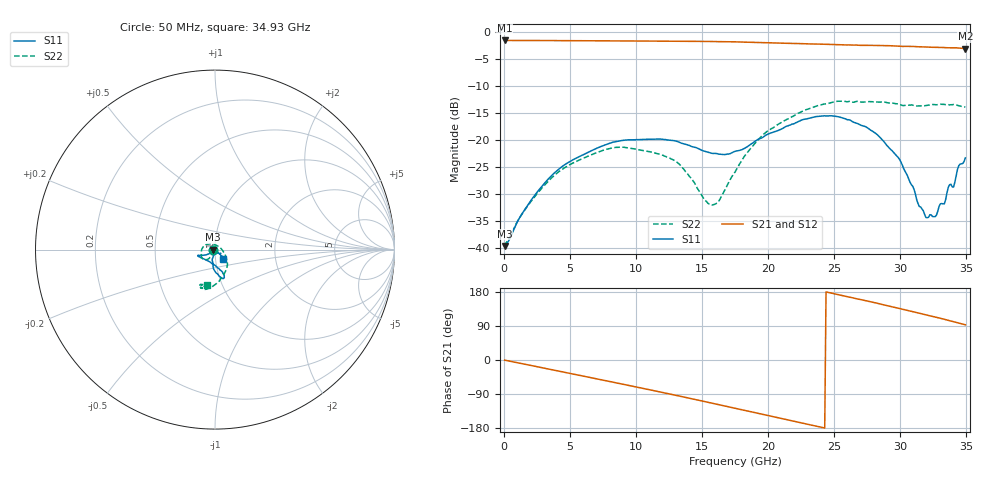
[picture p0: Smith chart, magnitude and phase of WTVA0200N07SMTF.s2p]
! 50 ohm 2-Port S-parameters measured by Modelithics Inc support@modelithics.com  Tampa, FL USA 813-866-6335 (February 2024)
! Smiths Interconnect,  2dB P/N: WTVA0200N07SMTF, Temperature: 50 C
! Board: 10 mil Rogers 4350B, Mounting Pad Dimensions: Length: 15 mils, Width: 25 mils, Gap: 40 mils.
# Hz S RI R 50
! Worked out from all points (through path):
!   352 points, 50 MHz to 34.93 GHz, reference 50 ohm
!   highest |S21| = -1.60 dB at 50 MHz (marker M1); lowest = -3.1 dB at 34.93 GHz (marker M2)
!   group delay of S21, straight-line fit = 21.1 ps
!   lowest |S11| = -39.5 dB at 50 MHz (marker M3), VSWR 1.02, Z = 49 - j0.000565 ohm
!   |S11| at or under -10 dB: start of sweep to end of sweep
!   |S22| runs from -39.6 to -12.8 dB; largest |S21 - S12| = 0.008
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5e7  -0.0106 -5.77e-06  0.8321 -0.00491  0.8316 -0.00493  -0.0105 -0.000887
1.2945e9  -0.0167 -0.0114  0.821 -0.1317  0.8206 -0.1317  -0.0142 -0.0143
2.986e9  -0.0318 -0.0223  0.7752 -0.2987  0.7745 -0.299  -0.0203 -0.0314
5.8715e9  -0.0651 -0.0313  0.6192 -0.549  0.6187 -0.5487  -0.0398 -0.0537
8.6575e9  -0.0926 -0.0319  0.3938 -0.723  0.3928 -0.7229  -0.0715 -0.0479
1.1742e10  -0.0963 -0.0348  0.0888 -0.8153  0.0875 -0.8147  -0.0744 -0.000362
1.3334e10  -0.0859 -0.0402  -0.0789 -0.8154  -0.0802 -0.8146  -0.0526 0.0269
1.56225e10  -0.051 -0.0568  -0.3176 -0.7493  -0.3185 -0.748  0.00827 0.0238
1.62195e10  -0.0419 -0.0614  -0.3753 -0.7197  -0.3754 -0.7189  0.0226 0.0147
1.7513e10  -0.0195 -0.0765  -0.4911 -0.6416  -0.4907 -0.641  0.0488 -0.0158
1.98015e10  0.0236 -0.108  -0.652 -0.4548  -0.6515 -0.4544  0.0673 -0.0962
2.33835e10  0.0521 -0.1537  -0.7665 -0.1014  -0.7658 -0.1017  -0.00708 -0.2001
2.61695e10  0.0269 -0.1512  -0.7324 0.1866  -0.7314 0.1881  -0.0738 -0.2158
2.91545e10  -0.0114 -0.084  -0.5868 0.458  -0.5826 0.4622  -0.0854 -0.203
2.99505e10  -0.0144 -0.0645  -0.5234 0.5183  -0.5209 0.5198  -0.0841 -0.197
3.1443e10  -0.00303 -0.0242  -0.3998 0.6066  -0.3973 0.6073  -0.067 -0.196
3.204e10  0.0043 -0.0187  -0.3429 0.6363  -0.3409 0.6366  -0.0605 -0.2007
3.33335e10  0.0187 -0.0179  -0.2128 0.6834  -0.2095 0.6837  -0.0592 -0.2054
3.3632e10  0.0278 -0.024  -0.1824 0.6883  -0.1771 0.6891  -0.0562 -0.2049
3.403e10  0.0293 -0.0225  -0.1412 0.6972  -0.136 0.6975  -0.0544 -0.2065
3.4428e10  0.0433 -0.0388  -0.0906 0.7022  -0.0899 0.7016  -0.0522 -0.2011
3.49255e10  0.0457 -0.0511  -0.0355 0.6993  -0.0361 0.6985  -0.0435 -0.1981
